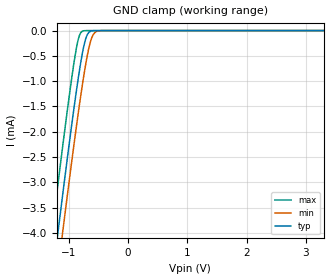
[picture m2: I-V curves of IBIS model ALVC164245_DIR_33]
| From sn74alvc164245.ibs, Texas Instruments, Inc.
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[Model]   ALVC164245_DIR_33
Model_type  Input
Vinl=0.8
Vinh=2
| variable   typ   min   max
C_comp   6.5pF   NA   NA
[Temperature Range]   40   100   -40
| Ambient temperature   25   85   -40
[Voltage range]   3.3   3   3.6
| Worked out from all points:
|   GND clamp passes 1 mA (typ) near -0.85 V on its own axis
[GND Clamp]
| ALVC164245_DIR_33
|   Voltage   I(typ)   I(min)   I(max)
-3.3V     -24.83mA   -25.52mA   -23.96mA
-1.3V     -5.111mA   -5.849mA   -4.158mA
-1.26V    -4.729mA   -5.468mA   -3.775mA
-1.185V   -4.018mA   -4.758mA   -3.062mA
-1.09V    -3.13mA    -3.869mA   -2.175mA
-880mV    -1.265mA   -1.975mA   -406.2uA
-825mV    -828.8uA   -1.509mA   -114.4uA
-770mV    -446.6uA   -1.069mA   -12.88uA
-700mV    -116.1uA   -571.7uA   -455.3nA
-630mV    -13.33uA   -205.5uA   -15.19nA
-500mV    -126.5nA   -7.204uA   -35.76pA
3.3V      6.303pA    16.94nA    5.63pA
